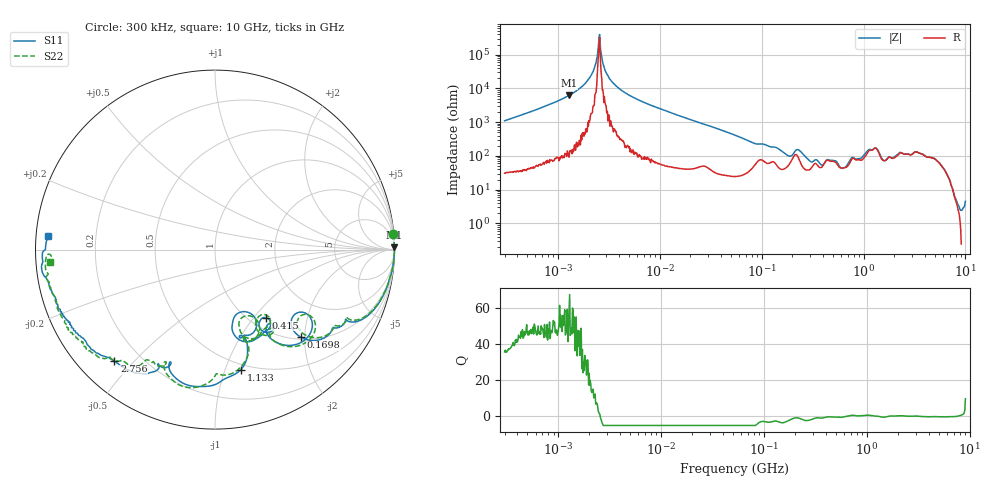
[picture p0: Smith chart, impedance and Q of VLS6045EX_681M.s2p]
! S-Parameter Data Generated by TDK Corporation
! Copyright(C) 2019 TDK Corporation.
! All Rights Reserved.
! TDK P/N: VLS6045EX-681M (Inductor)
! Property: L=680uH at 100kHz
! Size(LxWxT): 6x6x4.5mm
! Model Type: s2p (Touchstone File Format Version 1.0)
! Frequency: DC=Yes Start=0.3MHz Stop=10000MHz 802points Log-sweep
! Model Generated on May 10, 2019
! Port Assignments:
!  1 ---@@@--- 2
! Applicable Conditions:
!  Temperature = 25 degC
!  DC Bias Current = 0 A
!  Small Signal Operation
! Terms and conditions regarding TDK Simulation Models
! (1)This simulation model is being provided solely for informational purposes. Please refer to the specifications of the products in terms of detailed characteristics of such products.
! (2)In no event shall TDK Corporation of any of its subsidiaries be liable for any loss or damage arising, directly or indirectly,
!  From any information contained in this simulation model, including, but not limited to loss or damages arising from any inaccuracies, omissions or errors in connection with such information.
! (3)Any and all copyrights on this simulation model are owned by TDK Corporation.
!  Duplication or redistribution of this simulation model without prior written permission from TDK Corporation is prohibited.
! (4)This simulation model is subject to any modification or change without any prior notice.
! (5)Neither TDK Corporation nor any of its subsidiaries shall make any warranty, express or implied,
!  Including but not limited to the correctness, implied warranties of merchantability and fitness for a particular purpose with respect to this simulation models.
! (6)The use of this simulation model shall be deemed to have consented to the terms and conditions hereof.
# Hz S MA R 50
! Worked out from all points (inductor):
!   801 points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, 300 kHz to 10 GHz, reference 50 ohm
!   read as one part in series: L = 575 uH near 318.3 kHz
!   highest Q = 55.2 at 1.288 MHz (marker M1), where L = 768 uH
!   self-resonance near 2.534 MHz
!   S11 on the Smith chart (normalised r, x): 300 kHz: 2, +23; 169.8 MHz: 1.05, -1.91; 415 MHz: 1.18, -1.16; 1.133 GHz: 0.45, -1.13; 2.756 GHz: 0.11, -0.44; 10 GHz: 0.04, +0.04
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300000  0.9932 5.0  0.09012 -83.4  0.09018 -83.4  0.993 4.9
1288123  0.9996 0.8  0.01608 -88.4  0.01605 -88.1  0.9996 0.8
1713600  0.9997 0.3  0.008929 -88.1  0.008932 -88.2  0.9997 0.3
2178889  0.9997 -0.0  0.003462 -86.2  0.00351 -85.5  0.9997 0.0
2566584  0.9997 -0.3  0.0002516 34.2  0.0003245 22.1  0.9997 -0.2
2889664  0.9997 -0.4  0.002743 83.3  0.002719 84.1  0.9997 -0.4
3553821  0.9997 -0.8  0.00732 86.6  0.007343 86.8  0.9996 -0.7
9671944  0.9983 -3.1  0.03826 85.6  0.03827 85.7  0.9984 -3.0
5.477226e7  0.9598 -18.2  0.2296 68.7  0.2296 68.7  0.9599 -17.7
1.69821e8  0.6822 -45.6  0.5292 26.2  0.5293 26.2  0.6984 -43.2
2.013356e8  0.5768 -37.7  0.4877 7.7  0.4877 7.7  0.6084 -36.7
2.289088e8  0.7012 -39.9  0.416 17.4  0.416 17.4  0.7208 -39.9
3.126428e8  0.5147 -56.1  0.601 -0.3  0.6011 -0.3  0.5408 -56.0
4.149731e8  0.4734 -53.1  0.5726 -19.0  0.5726 -19.0  0.453 -52.9
5.414944e8  0.5483 -69.3  0.5294 -20.0  0.5294 -20.1  0.5416 -63.9
7.069847e8  0.3867 -63.6  0.5914 -50.4  0.5914 -50.4  0.4111 -63.5
1.133369e9  0.6836 -77.8  0.2785 -82.7  0.2784 -82.7  0.699 -83.0
1.43752e9  0.7589 -105.1  0.2424 -60.7  0.2423 -60.8  0.7789 -105.1
1.767019e9  0.7028 -111.8  0.2602 -93.3  0.26 -93.3  0.7083 -114.1
2.756092e9  0.8371 -132.1  0.1292 -114.6  0.1292 -114.6  0.8346 -132.1
5.284132e9  0.9242 -158.9  0.05732 -123.5  0.0573 -123.6  0.9264 -153.1
1e10  0.9318 175.4  0.05495 -147.1  0.05473 -146.8  0.9194 -175.8
